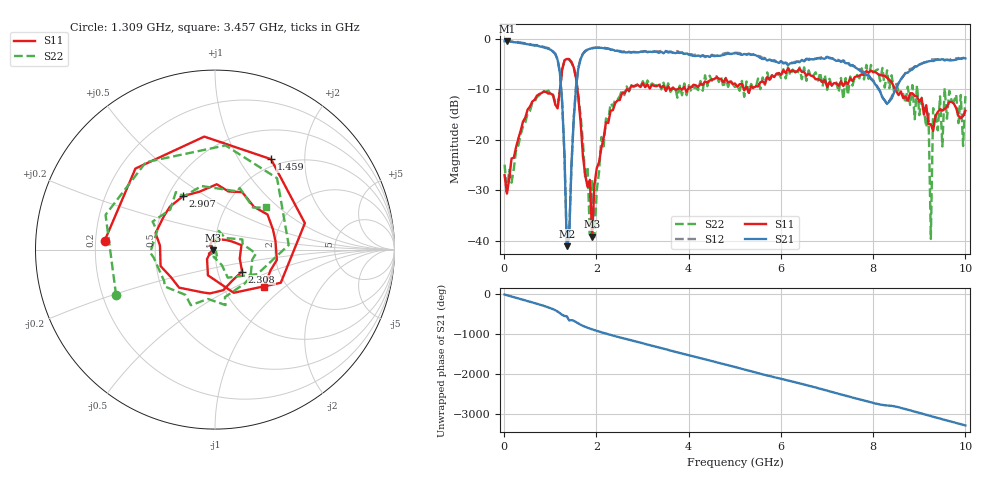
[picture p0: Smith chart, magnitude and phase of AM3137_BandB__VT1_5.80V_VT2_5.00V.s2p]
! Date/Time: Tue, Nov 13, 2018 4:52 PM
! Network Analyzer: Agilent Technologies E8364B Rev: A.07.50.67
! Sweep from 0.010 to 10.000 GHz, 201 Points, Sweep Type: LIN
! Power Supply: 5.801 V, 0.002 A
# Hz S DB R 50
!freq MagS11 AngS11 MagS21 AngS21 MagS12 AngS12 MagS22 AngS22
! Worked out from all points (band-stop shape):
!   201 points, 10 MHz to 10 GHz, reference 50 ohm
!   highest |S21| = -0.43 dB at 59.95 MHz (marker M1); lowest = -41.1 dB at 1.359 GHz (marker M2)
!   |S21| within 3 dB of the highest: start of sweep to 1.129 GHz; 1.684 GHz to 4.254 GHz (2.57 GHz wide, 86.6 % of centre)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
!   lowest |S11| = -39.2 dB at 1.908 GHz (marker M3), VSWR 1.02, Z = 49 - j0.352 ohm
!   |S11| at or under -10 dB: start of sweep to 1.212 GHz; 1.588 GHz to 2.656 GHz (1.069 GHz wide, 50.4 % of centre); 8.48 GHz to end of sweep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
!   |S22| runs from -39.7 to -3.9 dB; largest |S21 - S12| = 0.035
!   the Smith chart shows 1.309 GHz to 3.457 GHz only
!   S11 on the Smith chart (normalised r, x): 1.309 GHz: 0.24, +0.04; 1.459 GHz: 0.89, +1.39; 2.308 GHz: 1.31, -0.33; 2.907 GHz: 0.60, +0.41; 3.457 GHz: 1.54, -0.73
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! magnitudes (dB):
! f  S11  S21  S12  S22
! 10 MHz  -27.0  -0.5  -0.3  -24.9
! 59.95 MHz  -30.7  -0.4  -0.3  -30.4
! 1.109 GHz  -13.0  -3.0  -2.9  -12.7
! 1.309 GHz  -4.2  -23.3  -23.2  -4.3
! 1.359 GHz  -4.0  -41.1  -41.0  -3.9
! 1.459 GHz  -4.5  -25.3  -25.2  -4.7
! 1.708 GHz  -23.3  -3.0  -2.9  -20.5
! 1.858 GHz  -27.9  -1.9  -1.9  -38.8
! 1.908 GHz  -39.2  -1.8  -1.8  -27.9
! 1.958 GHz  -28.9  -1.8  -1.7  -39.3
! 2.308 GHz  -14.2  -2.2  -2.1  -12.8
! 2.907 GHz  -9.2  -2.7  -2.5  -8.8
! 3.357 GHz  -9.1  -2.7  -2.5  -8.6
! 3.457 GHz  -9.3  -2.8  -2.4  -8.7
! 5.005 GHz  -8.8  -2.8  -2.7  -9.5
! 6.703 GHz  -7.4  -4.1  -3.9  -7.2
! 8.352 GHz  -8.1  -12.4  -12.3  -9.8
! 9.201 GHz  -16.9  -4.4  -4.3  -14.8
! 9.251 GHz  -16.9  -4.4  -4.1  -39.7
! 9.301 GHz  -18.2  -4.4  -4.1  -13.7
! 9.95 GHz  -15.3  -3.7  -3.8  -21.2
! 10 GHz  -14.2  -3.9  -3.7  -11.3
